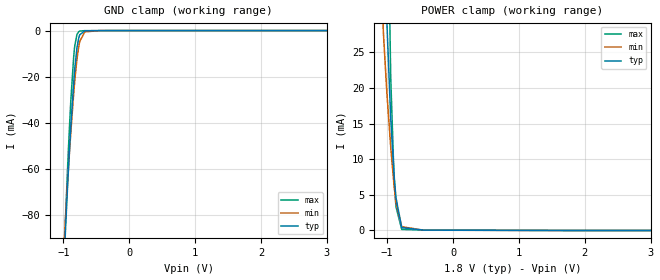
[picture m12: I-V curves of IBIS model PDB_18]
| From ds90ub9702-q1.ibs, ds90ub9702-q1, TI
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|   PDB_18 Model
[Model]   PDB_18
Model_type   Input
Vinl = 0.63
Vinh = 1.17
|   typ   min   max
C_comp   1.157818pF   1.212384pF   1.105708pF
[Voltage Range]   1.8   1.71   1.89
[Temperature Range]   27   105   -40
[Power Clamp Reference]   1.8   1.71   1.89
[GND Clamp Reference]   0   0   0
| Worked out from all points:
|   GND clamp passes 1 mA (typ) near -0.72 V on its own axis
|   POWER clamp passes 1 mA (typ) near -0.79 V on its own axis
[GND Clamp]
|   Voltage   I(typ)   I(min)   I(max)
-1.8V     -703.7mA   -630.8mA   -757.8mA
-1.001V   -105.8mA   -97.23mA   -103.4mA
-936mV    -66.54mA   -65.2mA    -58.66mA
-909mV    -51.9mA    -52.97mA   -42.02mA
-887.4mV  -41.08mA   -43.73mA   -30.02mA
-844.2mV  -22.31mA   -27.07mA   -11.24mA
-828mV    -16.51mA   -21.62mA   -6.629mA
-795.6mV  -7.606mA   -12.49mA   -1.734mA
-757.8mV  -2.233mA   -5.419mA   -298.2uA
-676.8mV  -107.1uA   -556.7uA   -27.88uA
-444.6mV  -13.4uA    -11.66uA   -16.36uA
3.6V      0A         0A         0A
[POWER Clamp]
|   Voltage   I(typ)   I(min)   I(max)
-1.8V     913.3mA    660mA      1.143A
-1.076V   62.45mA    31.28mA    126.5mA
-1.055V   49.98mA    27.29mA    103mA
-1.012V   31.67mA    20.37mA    61.71mA
-1.001V   28.27mA    18.81mA    53.01mA
-946.8mV  15.76mA    11.75mA    21.58mA
-898.2mV  8.218mA    6.547mA    7.957mA
-876.6mV  5.65mA     4.688mA    4.551mA
-865.8mV  4.553mA    3.883mA    3.294mA
-779.4mV  397.2uA    529.1uA    150.7uA
-444.6mV  44.91uA    37.41uA    55.69uA
3.6V      0A         0A         0A
